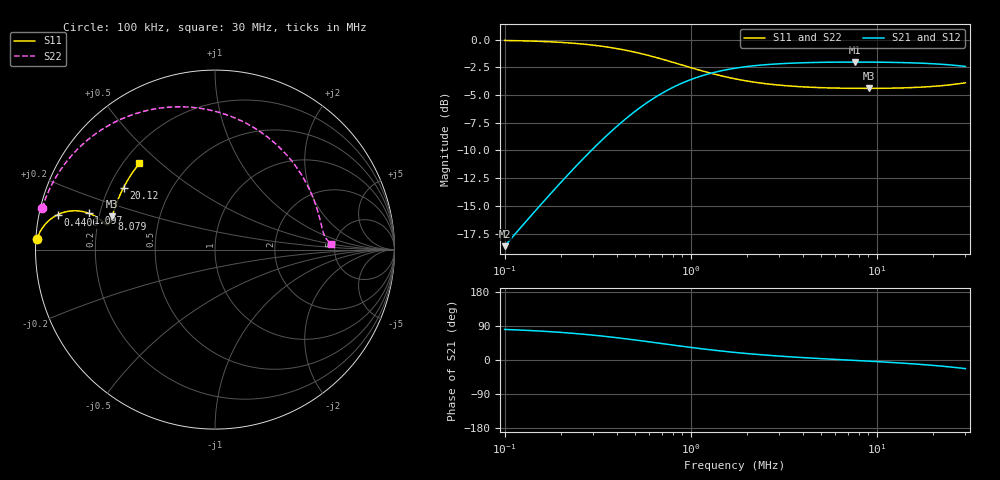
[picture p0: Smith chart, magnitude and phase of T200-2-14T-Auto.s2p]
! ListType=Log
!!T200-2 14T 4:1 Z ratio Auto-Transformer
# MHZ S RI R 50
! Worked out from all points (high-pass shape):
!   101 points, 100 kHz to 30 MHz, reference 50 ohm
!   highest |S21| = -2.02 dB at 7.632 MHz (marker M1); lowest = -18.6 dB at 100 kHz (marker M2)
!   |S21| within 3 dB of the highest: 672.3 kHz to end of sweep
!   lowest |S11| = -4.4 dB at 9.056 MHz (marker M3), VSWR 4.03, Z = 12.7 + j7.43 ohm
!   |S11| at or under -10 dB: nowhere
!   |S22| runs from -4.3 to -0.1 dB; largest |S21 - S12| = 0.0027
!   S11 on the Smith chart (normalised r, x): 100 kHz: 0.00, +0.03; 440.6 kHz: 0.05, +0.11; 1.097 MHz: 0.16, +0.14; 8.079 MHz: 0.25, +0.14; 20.12 MHz: 0.26, +0.29; 30 MHz: 0.26, +0.43
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0.1  -0.99 0.0611  0.019 0.1154  0.019 0.1153  -0.9629 0.2306
0.1330014  -0.9834 0.0799  0.0319 0.1508  0.0319 0.1507  -0.9374 0.3014
0.1768936  -0.9724 0.1032  0.0535 0.1946  0.0535 0.1946  -0.8947 0.3892
0.2222271  -0.9586 0.125  0.0804 0.2355  0.0804 0.2354  -0.8415 0.4712
0.2637003  -0.9445 0.1427  0.1081 0.2685  0.108 0.2684  -0.7868 0.5374
0.350725  -0.912 0.1727  0.172 0.3236  0.172 0.3235  -0.6604 0.6487
0.4406071  -0.8771 0.194  0.2406 0.3616  0.2406 0.3615  -0.5246 0.7262
0.5535239  -0.8352 0.2095  0.323 0.3868  0.323 0.3867  -0.3614 0.779
0.6953784  -0.7894 0.2162  0.4132 0.3935  0.4132 0.3933  -0.1827 0.7957
0.8735868  -0.744 0.2133  0.5026 0.3794  0.5026 0.3792  -0.00556 0.7723
1.097466  -0.7031 0.2023  0.5827 0.3473  0.5827 0.3471  0.1534 0.7142
1.378719  -0.6695 0.1866  0.6484 0.3033  0.6483 0.303  0.2839 0.6339
1.833715  -0.6384 0.166  0.7085 0.2414  0.7083 0.2411  0.4038 0.5222
2.175933  -0.6249 0.1552  0.7341 0.2043  0.7339 0.204  0.4552 0.4569
2.733571  -0.6114 0.1443  0.7585 0.1573  0.7582 0.157  0.5049 0.3769
4.567423  -0.5929 0.1398  0.7861 0.0651  0.7858 0.0647  0.5651 0.2365
7.631539  -0.579 0.1684  0.7922 -0.0153  0.7917 -0.016  0.5901 0.1463
8.079479  -0.5771 0.1739  0.7919 -0.0242  0.7914 -0.0249  0.5919 0.1387
9.055779  -0.5731 0.1865  0.7909 -0.0422  0.7903 -0.0429  0.5953 0.1248
12.04431  -0.5593 0.2282  0.7847 -0.0896  0.7839 -0.0904  0.6032 0.096
20.12439  -0.5092 0.3458  0.7544 -0.1919  0.7529 -0.1928  0.6213 0.0587
30  -0.4212 0.4799  0.6984 -0.293  0.6958 -0.2937  0.6489 0.0307
